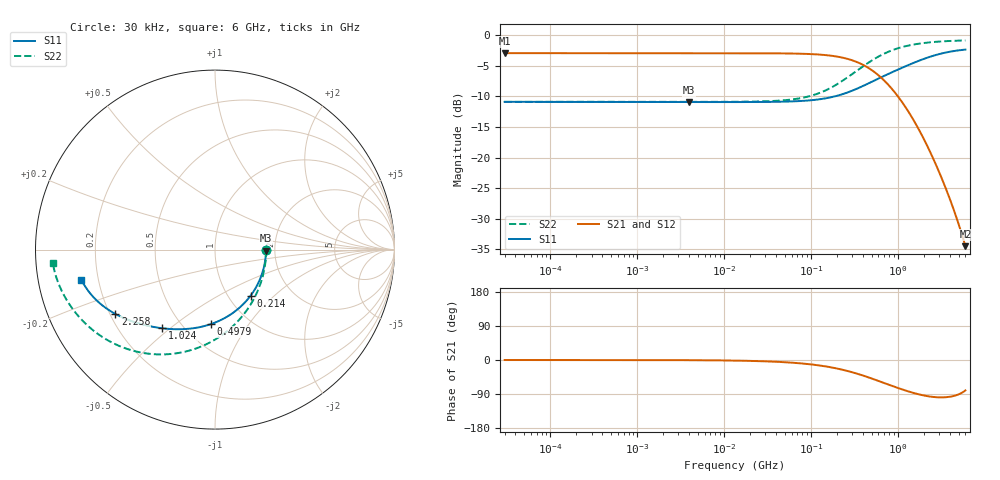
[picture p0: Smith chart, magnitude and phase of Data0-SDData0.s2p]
!EMIF06-MSD04F3
!Simulation
!24/03/11  09:12
!Start Freq. :30.000kHz; Stop Freq. : 6.000GHz
!Number of points : 1592; Sweep : LOGARITHMIC
!A1-A4 (Data0-SDData0)
!Freq ReS11 ImS11 ReS21 ImS21 ReS12 ImS12 ReS22 ImS22
# Hz  S  RI  R  50
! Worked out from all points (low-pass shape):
!   1592 points, 30 kHz to 6 GHz, reference 50 ohm
!   highest |S21| = -2.92 dB at 30 kHz (marker M1); lowest = -34.5 dB at 6 GHz (marker M2)
!   |S21| within 3 dB of the highest: start of sweep to 528.6 MHz
!   lowest |S11| = -10.9 dB at 3.955 MHz (marker M3), VSWR 1.79, Z = 89.7 - j1.05 ohm
!   |S11| at or under -10 dB: start of sweep to 187.8 MHz
!   |S22| runs from -10.9 to -0.9 dB; largest |S21 - S12| = 2e-15
!   S11 on the Smith chart (normalised r, x): 30 kHz: 1.80, -0.00; 214 MHz: 1.26, -0.72; 497.9 MHz: 0.68, -0.68; 1.024 GHz: 0.39, -0.47; 2.258 GHz: 0.22, -0.28; 6 GHz: 0.14, -0.11
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30000  0.2855 -0.000524  0.7142 -0.000312  0.7142 -0.000312  0.2857 -0.000211
231093.6  0.2844 -0.000816  0.7135 -0.000615  0.7135 -0.000615  0.2853 -0.000631
1766531  0.2841 -0.00251  0.7134 -0.00264  0.7134 -0.00264  0.2852 -0.00367
3954770  0.2841 -0.00539  0.7133 -0.00577  0.7133 -0.00577  0.2852 -0.00815
1.350376e7  0.2837 -0.0182  0.7129 -0.0196  0.7129 -0.0196  0.2845 -0.0277
4.336319e7  0.2801 -0.058  0.7084 -0.0624  0.7084 -0.0624  0.2784 -0.0885
6.820056e7  0.2743 -0.0905  0.7011 -0.0973  0.7011 -0.0973  0.2686 -0.1381
1.032257e8  0.2622 -0.1348  0.6859 -0.1444  0.6859 -0.1444  0.2479 -0.2052
1.538584e8  0.2372 -0.1944  0.6547 -0.2067  0.6547 -0.2067  0.2055 -0.2943
2.140201e8  0.1986 -0.2564  0.6067 -0.2691  0.6067 -0.2691  0.1403 -0.3847
3.214558e8  0.1163 -0.3404  0.5061 -0.346  0.5061 -0.346  0.00269 -0.4998
4.046889e8  0.0497 -0.3837  0.4266 -0.3776  0.4266 -0.3776  -0.1067 -0.5512
4.978761e8  -0.021 -0.4145  0.3449 -0.3907  0.3449 -0.3907  -0.2203 -0.5786
6.219965e8  -0.1042 -0.4357  0.2538 -0.3842  0.2538 -0.3842  -0.3491 -0.5821
7.890804e8  -0.1956 -0.4438  0.1631 -0.3537  0.1631 -0.3537  -0.4815 -0.556
1.024365e9  -0.2931 -0.4384  0.083 -0.2994  0.083 -0.2994  -0.6066 -0.4998
1.492066e9  -0.4244 -0.4115  0.0129 -0.2067  0.0129 -0.2067  -0.7386 -0.3953
2.258333e9  -0.5549 -0.3588  -0.0121 -0.1181  -0.0121 -0.1181  -0.8264 -0.2807
2.931712e9  -0.6248 -0.313  -0.0117 -0.0779  -0.0117 -0.0779  -0.86 -0.2169
3.747899e9  -0.6781 -0.2639  -0.00692 -0.0508  -0.00692 -0.0508  -0.8813 -0.1634
4.575669e9  -0.7119 -0.2223  -0.00235 -0.0347  -0.00235 -0.0347  -0.8931 -0.1243
6e9  -0.7452 -0.1671  0.0032 -0.0186  0.0032 -0.0186  -0.9034 -0.0763
